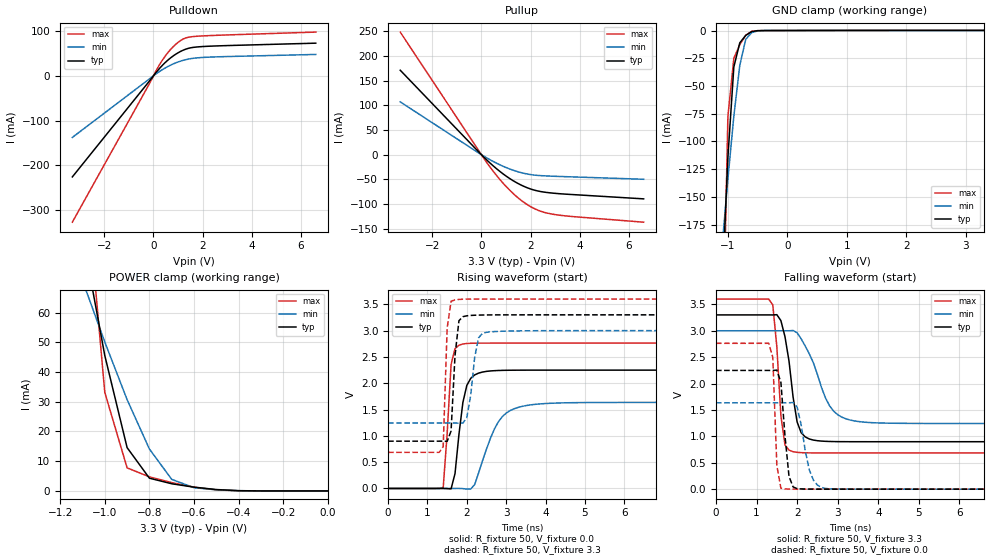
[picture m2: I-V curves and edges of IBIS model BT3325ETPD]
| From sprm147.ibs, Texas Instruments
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[Model]   BT3325ETPD
Model_type   I/O
Vinh = 2.00
Vinl = 0.80
Enable   Active-Low
Polarity   Non-Inverting
| signals   A, GZ, Y
Vmeas = 1.5
|   typ   min   max
C_comp   1.3959579p   1.3603035p   1.4235673p
|   typ   min   max
[Temperature Range]   25   -40   125
|   typ   min   max
[Voltage Range]   3.30V   3.00V   3.60V
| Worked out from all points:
|   slope of the pulldown table from 0 to 0.495 V, typ, clamps not added: 16.2 ohm
|   slope of the pullup table from 0 to 0.495 V, typ, clamps not added: 21.2 ohm
|   GND clamp passes 1 mA (typ) near -0.60 V on its own axis
|   POWER clamp passes 1 mA (typ) near -0.57 V on its own axis
|   rising waveform, R_fixture 50, V_fixture 0.0: 20-80 % time 228ps typ, 531ps min, 136ps max; typ from 0 V to 2.25 V
|   falling waveform, R_fixture 50, V_fixture 3.3: 20-80 % time 262ps typ, 547ps min, 162ps max; typ from 3.3 V to 0.899 V
|   rising waveform, R_fixture 50, V_fixture 3.3: 20-80 % time 124ps typ, 184ps min, 77.8ps max; typ from 0.899 V to 3.3 V
|   falling waveform, R_fixture 50, V_fixture 0.0: 20-80 % time 151ps typ, 247ps min, 80.8ps max; typ from 2.25 V to 0 V
[Pulldown]
|   Voltage   I(typ)   I(min)   I(max)
-3.3V     -226mA     -137.8mA   -327.2mA
-200mV    -14.16mA   -8.386mA   -21.14mA
200mV     13.61mA    7.952mA    20.54mA
400mV     25.49mA    15.02mA    38.03mA
600mV     35.71mA    21.19mA    52.74mA
1V        51.44mA    30.9mA     74.72mA
1.3V      59.31mA    35.9mA     84.44mA
1.7V      64.08mA    39.68mA    88.13mA
6.6V      72.96mA    47.76mA    97.72mA
[GND_clamp]
|   Voltage   I(typ)   I(min)   I(max)
-3.3V     -3.511A    -1.718A    -9.218A
-1.1V     -235.8mA   -196.1mA   -330.1mA
-1V       -114.6mA   -134.2mA   -77.7mA
-900mV    -32.86mA   -77.3mA    -25.01mA
-800mV    -11.1mA    -31.4mA    -12.76mA
-700mV    -4.361mA   -7.942mA   -4.34mA
-600mV    -997uA     -1.899mA   -689.8uA
-500mV    -141.7uA   -368.6uA   -107.4uA
-400mV    -41.6uA    -63.91uA   -57.91uA
3.3V      101.5uA    62.96uA    182uA
[Pullup]
|   Voltage   I(typ)   I(min)   I(max)
-3.3V     171mA      106.9mA    248.3mA
300mV     -14.55mA   -8.884mA   -21.5mA
700mV     -31.87mA   -19.32mA   -47.22mA
1V        -43.2mA    -26mA      -64.19mA
1.6V      -61.21mA   -36.17mA   -91.8mA
1.9V      -67.72mA   -39.52mA   -102.3mA
2.2V      -72.46mA   -41.63mA   -110.4mA
2.5V      -75.47mA   -42.73mA   -116.1mA
2.9V      -77.9mA    -43.66mA   -120.6mA
3.7V      -80.82mA   -45.04mA   -125.3mA
6.6V      -89.55mA   -49.85mA   -136.8mA
[POWER_clamp]
|   Voltage   I(typ)   I(min)   I(max)
-3.3V     1.142A     572.3mA    2.729A
-1.1V     86.16mA    70.78mA    117.7mA
-1V       45.58mA    50.11mA    33.16mA
-900mV    14.58mA    30.72mA    7.765mA
-800mV    4.282mA    14.1mA     4.743mA
-700mV    2.41mA     3.892mA    2.788mA
-600mV    1.264mA    1.078mA    1.296mA
-500mV    464.6uA    368.9uA    356.7uA
-400mV    81.42uA    82.49uA    33.99uA
0V        1pA        1pA        1pA
[Ramp]
|   I(typ)   I(min)   I(max)
dV/dt_r   1.349/0.218n   0.981/0.526n   1.658/0.107n
dV/dt_f   1.441/0.253n   1.053/0.543n   1.748/0.140n
[Rising Waveform]
R_fixture = 50
V_fixture = 0.0
|  pu_on
|  TIME   V(typ)   V(min)   V(max)
0s        15nV       177nV      1nV
1.4ns     463.3uV    -1.125uV   13.85mV
1.6ns     -7.836mV   -4.528uV   2.353V
1.7ns     281.8mV    322.1uV    2.656V
1.8ns     1.027V     950.6uV    2.723V
1.9ns     1.635V     -3.61mV    2.746V
2.1ns     2.094V     -9.588mV   2.759V
2.8ns     2.242V     1.266V     2.763V
3.3ns     2.248V     1.54V      2.763V
10ns      2.249V     1.636V     2.763V
[Falling Waveform]
R_fixture = 50
V_fixture = 3.3
V_fixture_min = 3.0
V_fixture_max = 3.6
|  pd_on
|  TIME   V(typ)   V(min)   V(max)
0s        3.3V       3V         3.6V
1.4ns     3.299V     3V         3.49V
1.5ns     3.304V     3V         2.697V
1.6ns     3.192V     3V         1.389V
1.7ns     2.89V      2.999V     839.3mV
1.9ns     1.747V     3.005V     709.5mV
2.2ns     989.6mV    2.71V      688.7mV
2.8ns     903.3mV    1.578V     686.2mV
3.3ns     898.9mV    1.31V      686.2mV
10ns      898.6mV    1.244V     686.2mV
[Rising Waveform]
R_fixture = 50
V_fixture = 3.3
V_fixture_min = 3.0
V_fixture_max = 3.6
|  pd_off
|  TIME   V(typ)   V(min)   V(max)
0s        898.6mV    1.244V     686.2mV
1.4ns     898.9mV    1.244V     796.2mV
1.5ns     894.3mV    1.244V     3.044V
1.6ns     1.092V     1.245V     3.558V
1.7ns     2.525V     1.244V     3.585V
1.8ns     3.188V     1.24V      3.593V
1.9ns     3.266V     1.243V     3.597V
2.3ns     3.295V     2.865V     3.6V
2.4ns     3.297V     2.95V      3.6V
10ns      3.3V       3V         3.6V
[Falling Waveform]
R_fixture = 50
V_fixture = 0.0
|  pu_off
|  TIME   V(typ)   V(min)   V(max)
0s        2.249V     1.636V     2.763V
1.3ns     2.249V     1.636V     2.763V
1.4ns     2.248V     1.636V     2.5V
1.5ns     2.254V     1.635V     448.7mV
1.6ns     2.022V     1.635V     17.04mV
1.8ns     241.4mV    1.637V     2.274mV
2ns       9.591mV    1.554V     608.1uV
2.3ns     1.59mV     364.5mV    127.5uV
2.6ns     408.8uV    33.13mV    46.24uV
10ns      239nV      1.103uV    134nV
